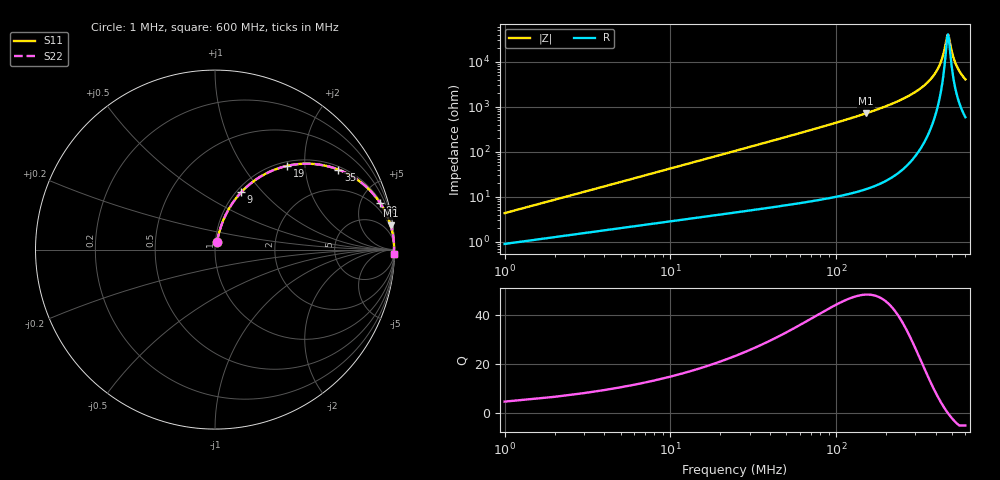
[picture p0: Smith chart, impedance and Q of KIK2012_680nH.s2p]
!version-2
!date-01.2022
!Series
# MHz S RI R 50
!Freq ReS11 ImS11 ReS21 ImS21 ReS12 ImS12 ReS22 ImS22
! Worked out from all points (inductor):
!   600 points, 1 MHz to 600 MHz, reference 50 ohm
!   read as one part in series: L = 680 nH near 4 MHz
!   highest Q = 48.4 at 151 MHz (marker M1), where L = 758 nH
!   self-resonance near 471 MHz
!   S11 on the Smith chart (normalised r, x): 1 MHz: 1.02, +0.09; 9 MHz: 1.05, +0.77; 19 MHz: 1.08, +1.63; 35 MHz: 1.11, +3.01; 80 MHz: 1.17, +7.04; 600 MHz: 13, -81
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1  0.0107 0.0419  0.9893 -0.0419  0.9893 -0.0419  0.0107 0.0419
5  0.061 0.1966  0.939 -0.1966  0.939 -0.1966  0.061 0.1966
7  0.1002 0.2629  0.8998 -0.2629  0.8998 -0.2629  0.1002 0.2629
9  0.1462 0.3198  0.8538 -0.3198  0.8538 -0.3198  0.1462 0.3198
13  0.2492 0.4042  0.7508 -0.4042  0.7508 -0.4042  0.2492 0.4042
19  0.4032 0.4668  0.5968 -0.4668  0.5968 -0.4668  0.4032 0.4668
35  0.6874 0.4459  0.3126 -0.4459  0.3126 -0.4459  0.6874 0.4459
53  0.8332 0.3584  0.1668 -0.3584  0.1668 -0.3584  0.8332 0.3584
80  0.9199 0.2594  0.0801 -0.2594  0.0801 -0.2594  0.9199 0.2594
101  0.9492 0.2087  0.0508 -0.2087  0.0508 -0.2087  0.9492 0.2087
151  0.9783 0.1356  0.0217 -0.1356  0.0217 -0.1356  0.9783 0.1356
201  0.989 0.094  0.011 -0.094  0.011 -0.094  0.989 0.094
301  0.9961 0.0457  0.00385 -0.0457  0.00385 -0.0457  0.9961 0.0457
359  0.9974 0.0272  0.00261 -0.0272  0.00261 -0.0272  0.9974 0.0272
401  0.9977 0.016  0.0023 -0.016  0.0023 -0.016  0.9977 0.016
436  0.9977 0.00766  0.00229 -0.00766  0.00229 -0.00766  0.9977 0.00766
469  0.9976 0.000451  0.00244 -0.000451  0.00244 -0.000451  0.9976 0.000451
476  0.9975 -0.00101  0.00249 0.00101  0.00249 0.00101  0.9975 -0.00101
501  0.9973 -0.00606  0.00271 0.00606  0.00271 0.00606  0.9973 -0.00606
518  0.9971 -0.00936  0.00289 0.00936  0.00289 0.00936  0.9971 -0.00936
540  0.9968 -0.0135  0.00316 0.0135  0.00316 0.0135  0.9968 -0.0135
600  0.9959 -0.024  0.00411 0.024  0.00411 0.024  0.9959 -0.024
